[IBIS Ver]   2.1
[File Name]   ixp4xx.ibs
[File Rev]   0.00
[Date]   10/04/2004
[Source]   From silicon level SPICE model at Intel Corporation.
[Notes]   The following information corresponds to the IXP4XX chip.
[Disclaimer]   This information is for modeling purposes only and is not
   guaranteed.
[Copyright]   Copyright 2003, Intel Corporation, All Rights Reserved.
[Component]   IXP4XX
[Manufacturer]  Intel Corporation
[Package]
|   typ   min   max
R_pkg   130.00mOhm   81.000mOhm   260.00mOhm
L_pkg   5.00nH   4.00nH   7.00nH
C_pkg   1.10pF   800.00fF   2.00pF
[PIN] signal_name model_name R_pin L_pin C_pin
A1   PCI_AD[27]   pci
A2   PCI_GNT_N[1]   pci
A3   PCI_GNT_N[3]   pci
A4   SDM_DATA[19]   sdrdat
A5   SDM_DATA[27]   sdrdat
A6   SDM_DATA[26]   sdrdat
A7   SDM_DATA[25]   sdrdat
A8   SDM_DATA[23]   sdrdat
A9   SDM_DATA[14]   sdrdat
A10   SDM_DATA[13]   sdrdat
A11   SDM_DATA[11]   sdrdat
A12   SDM_DATA[10]   sdrdat
A13   SDM_DATA[6]   sdrdat
A14   SDM_DATA[8]   sdrdat
A15   SDM_DQM[1]   sdrdat
A16   SDM_CS_N[0]   sdrdat
A17   SDM_CLKOUT   sdrclk
A18   SDM_RAS_N   sdrdat
A19   SDM_ADDR[12]   sdrdat
A20   SDM_ADDR[9]   sdrdat
A21   SDM_ADDR[8]   sdrdat
A22   SDM_ADDR[5]   sdrdat
A23   EX_RD_N   gpio16x
A24   EX_ADDR[1]   gpio16x
A25   EX_ADDR[3]   gpio16x
A26   EX_ADDR[5]   gpio16x
B1   PCI_AD[28]   pci
B3   PCI_GNT_N[2]   pci
B5   SDM_DATA[28]   sdrdat
B7   SDM_DATA[21]   sdrdat
B9   SDM_DATA[0]   sdrdat
B11   SDM_DATA[12]   sdrdat
B13   SDM_DATA[9]   sdrdat
B15   SDM_DQM[2]   sdrdat
B17   SDM_CKE   sdrdat
B19   SDM_ADDR[10]   sdrdat
B21   SDM_ADDR[1]   sdrdat
B23   EX_IOWAIT_N   gpio16x
B26   EX_ADDR[9]   gpio16x
C1   PCI_AD[26]   pci
C2   PCI_AD[30]   pci
C4   PCI_INTA_N   pciod
C6   SDM_DATA[18]   sdrdat
C9   SDM_DATA[24]   sdrdat
C11   SDM_DATA[2]   sdrdat
C12   SDM_DATA[4]   sdrdat
C14   SDM_DATA[7]   sdrdat
C15   SDM_DQM[3]   sdrdat
C17   SDM_CAS_N   sdrdat
C18   SDM_ADDR[11]   sdrdat
C20   SDM_ADDR[6]   sdrdat
C21   SDM_ADDR[2]   sdrdat
C23   EX_ADDR[0]   gpio16x
C24   EX_ADDR[4]   gpio16x
C25   EX_ADDR[7]   gpio16x
C26   EX_ADDR[13]   gpio16x
D1   PCI_AD[25]   pci
D3   PCI_AD[31]   pci
D5   PCI_SERR_N   pciod
D7   SDM_DATA[29]   sdrdat
D8   SDM_DATA[20]   sdrdat
D10   SDM_DATA[15]   sdrdat
D11   SDM_DATA[1]   sdrdat
D13   SDM_DATA[5]   sdrdat
D15   SDM_WE_N   sdrdat
D16   SDM_CS_N[1]   sdrdat
D17   SDM_BA[1]   sdrdat
D19   SDM_ADDR[0]   sdrdat
D22   EX_ALE   gpio16x
D24   EX_ADDR[6]   gpio16x
D26   EX_ADDR[17]   gpio16x
E1   PCI_AD[23]   pci
E3   PCI_REQ_N[2]   pci
E5   PCI_GNT_N[0]   pci
E6   SDM_DATA[16]   sdrdat
E8   SDM_DATA[30]   sdrdat
E10   SDM_DATA[22]   sdrdat
E12   SDM_DATA[3]   sdrdat
E14   SDM_DQM[0]   sdrdat
E16   SDM_BA[0]   sdrdat
E18   SDM_ADDR[7]   sdrdat
E20   SDM_ADDR[3]   sdrdat
E24   EX_ADDR[10]   gpio16x
E25   EX_ADDR[15]   gpio16x
E26   EX_ADDR[19]   gpio16x
F1   PCI_AD[20]   pci
F2   PCI_IDSEL   pci
F4   PCI_REQ_N[0]   pci
F7   SDM_DATA[31]   sdrdat
F9   SDM_DATA[17]   sdrdat
F18   SDM_ADDR[4]   sdrdat
F22   EX_WR_N   gpio16x
F24   EX_ADDR[14]   gpio16x
F26   EX_ADDR[21]   gpio16x
G1   PCI_AD[21]   pci
G3   PCI_AD[24]   pci
G5   PCI_REQ_N[1]   pci
G21   EX_ADDR[2]   gpio16x
G23   EX_ADDR[12]   gpio16x
G25   EX_ADDR[20]   gpio16x
G26   EX_ADDR[22]   gpio16x
H1   PCI_AD[16]   pci
H2   PCI_AD[18]   pci
H4   PCI_CBE_N[3]   pci
H6   PCI_REQ_N[3]   pci
H22   EX_ADDR[11]   gpio16x
H23   EX_ADDR[18]   gpio16x
H26   EX_CS_N[1]   gpio6x
J1   PCI_CLKIN   pciclk
J4   PCI_AD[22]   pci
J6   PCI_AD[29]   pci
J21   EX_ADDR[8]   gpio16x
J22   EX_ADDR[16]   gpio16x
J24   EX_ADDR[23]   gpio16x
J25   EX_CS_N[2]   gpio6x
J26   EX_CS_N[4]   gpio6x
K1   PCI_CBE_N[2]   pci
K3   PCI_AD[17]   pci
K5   PCI_AD[19]   pci
K23   EX_CS_N[0]   gpio6x
K24   EX_CS_N[3]   gpio6x
K26   EX_CS_N[7]   gpio6x
L1   PCI_DEVSEL_N   pci
L3   PCI_STOP_N   pci
L5   PCI_FRAME_N   pci
L24   EX_CS_N[6]   gpio6x
L25   EX_DATA[0]   gpio16x
L26   EX_DATA[1]   gpio16x
M1   PCI_CBE_N[1]   pci
M2   PCI_PAR   pci
M4   PCI_IRDY_N   pci
M22   EX_CS_N[5]   gpio6x
M23   EX_CLK   gpio16x
M24   EX_DATA[2]   gpio16x
M26   EX_DATA[3]   gpio16x
N1   PCI_AD[11]   pci
N4   PCI_PERR_N   pci
N5   PCI_AD[15]   pci
N25   EX_DATA[4]   gpio16x
N26   EX_DATA[5]   gpio16x
U1   PCI_AD[8]   pci
U3   PCI_AD[0]   pci
U4   PCI_AD[7]   pci
U5   HSS_TXDATA0   gpio10x
U22   GPIO[14]   gpio6x
U23   EX_RDY_N[1]   gpio16x
U24   EX_RDY_N[2]   gpio16x
U25   GPIO[15]   gpio6x
U26   EX_DATA[15]   gpio16x
P1   PCI_CBE_N[0]   pci
P2   PCI_AD[14]   pci
P3   PCI_AD[13]   pci
P5   PCI_AD[12]   pci
P22   EX_DATA[6]   gpio16x
P23   EX_DATA[7]   gpio16x
P24   EX_DATA[8]   gpio16x
P26   EX_DATA[9]   gpio16x
R1   PCI_AD[10]   pci
R3   PCI_AD[9]   pci
R5   PCI_AD[4]   pci
R24   EX_DATA[12]   gpio16x
R25   EX_DATA[11]   gpio16x
R26   EX_DATA[10]   gpio16x
T1   PCI_AD[6]   pci
T2   PCI_TRDY_N   pci
T4   PCI_AD[2]   pci
T22   EX_RDY_N[0]   gpio16x
T24   EX_DATA[14]   gpio16x
T26   EX_DATA[13]   gpio16x
V1   PCI_AD[5]   pci
V3   PCI_AD[3]   pci
V5   HSS_TXFRAME0   gpio10x
V21   GPIO[6]   gpio9x
V22   GPIO[9]   gpio9x
V24   GPIO[13]   gpio9x
V26   EX_RDY_N[3]   gpio16x
W1   PCI_AD[1]   pci
W3   HSS_RXFRAME0   gpio10x
W5   HSS_TXCLK1   gpio10x
W6   HSS_RXFRAME1   gpio10x
W21   GPIO[1]   gpio9x
W23   GPIO[8]   gpio9x
W25   GPIO[11]   gpio9x
W26   GPIO[12]   gpio9x
Y1   HSS_TXCLK0   gpio10x
Y2   HSS_RXCLK0   gpio10x
Y3   HSS_TXFRAME1   gpio10x
Y6   ETH_TXEN0   gpio6x
Y21   RXDATA1   gpio6x
Y22   GPIO[0]   gpio9x
Y24   GPIO[5]   gpio9x
Y26   GPIO[10]   gpio9x
AA1   HSS_RXDATA0   gpio10x
AA4   HSS_RXCLK1   gpio10x
AA5   ETH_TXDATA0[2]  gpio6x
AA7   ETH_RXDATA0[1]  gpio6x
AA9   ETH_TXDATA1[1]  gpio6x
AA18   UTP_IP_FCI   gpio12x
AA19   UTP_IP_ADDR[0]  gpio12x
AA22   TXDATA1   gpio6x
AA24   GPIO[3]   gpio9x
AA26   GPIO[7]   gpio9x
AB1   HSS_TXDATA1   gpio10x
AB2   HSS_RXDATA1   gpio10x
AB3   ETH_TXDATA0[3]  gpio6x
AB4   ETH_TXDATA0[1]  gpio6x
AB6   ETH_RXCLK0   gpio6x
AB8   ETH_TXDATA1[2]  gpio6x
AB9   ETH_RXDATA1[1]  gpio6x
AB13   UTP_OP_DATA[7]  gpio12x
AB15   UTP_OP_SOC   gpio12x
AB17   UTP_IP_DATA[6]  gpio12x
AB19   UTP_IP_CLK   gpio12x
AB20   UTP_IP_ADDR[1]  gpio12x
AB21   SCANTESTMODE_N  gpio6x
AB23   CTS0_N   gpio6x
AB24   CTS1_N   gpio6x
AB26   GPIO[4]   gpio9x
AC2   ETH_TXDATA0[0]  gpio6x
AC5   ETH_RXDATA0[0]  gpio6x
AC8   ETH_RXDATA1[2]  gpio6x
AC13   RESET_IN_N   gpio6x
AC15   UTP_OP_DATA[1]  gpio12x
AC16   UTP_OP_FCI   gpio12x
AC17   UTP_OP_ADDR[1]  gpio12x
AC19   UTP_IP_DATA[2]  gpio12x
AC20   UTP_IP_SOC   gpio12x
AC22   JTG_TRST_N   gpio6x
AC24   RXDATA0   gpio6x
AC25   RTS1_N   gpio6x
AC26   GPIO[2]   gpio9x
AD1   ETH_TXCLK0   gpio6x
AD2   ETH_RXDV0   gpio6x
AD4   ETH_CRS0   gpio6x
AD5   ETH_MDC   gpio6x
AD6   ETH_TXDATA1[0]  gpio6x
AD7   ETH_RXDATA1[3]  gpio6x
AD8   ETH_RXCLK1   gpio6x
AD12   PLL_LOCK   gpio6x
AD14   UTP_OP_DATA[4]  gpio12x
AD15   UTP_OP_DATA[2]  gpio12x
AD17   UTP_OP_ADDR[3]  gpio12x
AD18   UTP_IP_DATA[7]  gpio12x
AD20   UTP_IP_DATA[1]  gpio12x
AD21   UTP_IP_ADDR[4]  gpio12x
AD23   JTG_TDO   gpio6x
AD25   TXDATA0   gpio6x
AD26   RTS0_N   gpio6x
AE1   ETH_RXDATA0[3]  gpio6x
AE3   ETH_COL0   gpio6x
AE4   ETH_TXEN1   gpio6x
AE6   ETH_RXDV1   gpio6x
AE8   ETH_COL1   gpio6x
AE14   UTP_OP_DATA[5]  gpio12x
AE16   UTP_OP_FCO   gpio12x
AE18   UTP_OP_ADDR[2]  gpio12x
AE20   UTP_IP_DATA[4]  gpio12x
AE22   UTP_IP_FCO   gpio12x
AE24   JTG_TDI   gpio6x
AE26   HIGHZ_N   gpio6x
AF1   ETH_RXDATA0[2]  gpio6x
AF2   ETH_MDIO   gpio6x
AF4   ETH_TXDATA1[3]  gpio6x
AF5   ETH_TXCLK1   gpio6x
AF6   ETH_RXDATA1[0]  gpio6x
AF7   ETH_CRS1   gpio6x
AF13   BYPASS_CLK   gpio6x
AF14   UTP_OP_DATA[6]  gpio12x
AF15   UTP_OP_DATA[3]  gpio12x
AF16   UTP_OP_DATA[0]  gpio12x
AF17   UTP_OP_CLK   gpio12x
AF18   UTP_OP_ADDR[4]  gpio12x
AF19   UTP_OP_ADDR[0]  gpio12x
AF20   UTP_IP_DATA[5]  gpio12x
AF21   UTP_IP_DATA[3]  gpio12x
AF22   UTP_IP_DATA[0]  gpio12x
AF23   UTP_IP_ADDR[3]  gpio12x
AF24   UTP_IP_ADDR[2]  gpio12x
AF25   JTG_TMS   gpio6x
AF26   JTG_TCK   gpio6x
| Models and submodels in the file (10): pci (I/O), pciclk (Input), sdrdat (I/O), sdrclk (I/O), gpio16x (I/O), pciod (I/O_open_drain), gpio6x (I/O), gpio10x (I/O), gpio9x (I/O), gpio12x (I/O)
